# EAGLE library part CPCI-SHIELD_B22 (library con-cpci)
Compact PCI - Abschirmblech unten B 22 / Lower Shield Type B 22 Source: www.erni.com
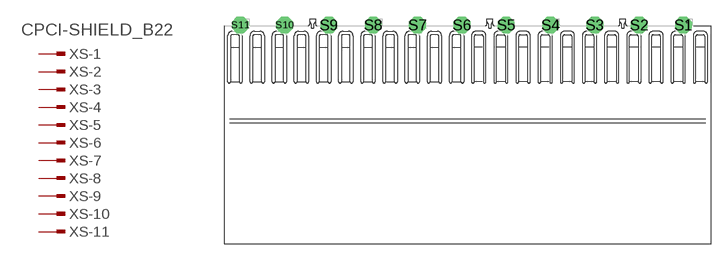
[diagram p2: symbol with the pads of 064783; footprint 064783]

Designator prefix XS; gates -1=PINV -2=PIN -3=PIN -4=PIN -5=PIN -6=PIN -7=PIN -8=PIN -9=PIN -10=PIN -11=PIN

## CPCI-SHIELD_B22 (OC_FARNELL: unknown; OC_NEWARK: unknown)  [064783]
S1  -1:1  in
S2  -2:1  in
S3  -3:1  in
S4  -4:1  in
S5  -5:1  in
S6  -6:1  in
S7  -7:1  in
S8  -8:1  in
S9  -9:1  in
S10  -10:1  in
S11  -11:1  in

## Footprint 064783 (pad centres in mm)
ERmet Abschirmblech unten B 22 / ERmet Lower Shield Type B 22 Source: http://www.erni.com/DB/PDF-Drawing/ERmet/064783.pdf
drill 1 octagon: S1 20,0; S2 16,0; S3 12,0; S4 8,0; S5 4,0; S6 0,0; S7 -4,0; S8 -8,0; S9 -12,0; S10 -16,0; S11 -20,0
